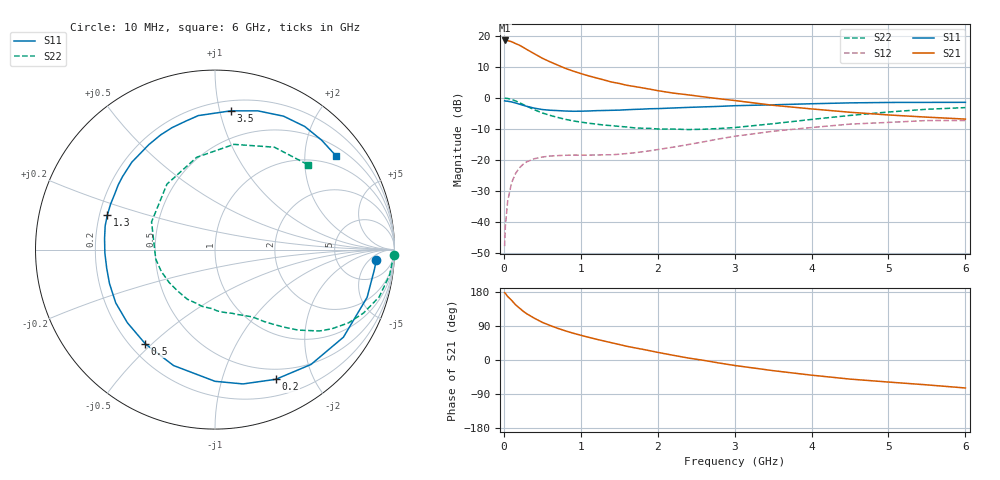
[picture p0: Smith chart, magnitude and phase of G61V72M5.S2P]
! SIEMENS Small Signal Semiconductors
! BFG193
! Si NPN RF Bipolar Junction Transistor in SOT223
! VCE = 1.75 V  IC = 2.5 mA
! Common Emitter S-Parameters:  August  1996
# GHz  S  MA  R  50
!  f  S11  S21  S12  S22
! GHz  MAG  ANG  MAG  ANG  MAG  ANG  MAG  ANG
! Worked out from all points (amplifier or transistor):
!   36 points, 10 MHz to 6 GHz, reference 50 ohm
!   highest |S21| = 18.6 dB at 10 MHz (marker M1)
!   |S21| within 3 dB of that: start of sweep to 305.1 MHz
!   unconditionally stable (mu >= 1): 1.312 GHz to 2.751 GHz
!   at 250 MHz: K = 0.21, MSG = 18.9 dB, |S12| = -21.4 dB
!   at 1.4 GHz: K = 1.07, MAG = 10.1 dB, |S12| = -18.3 dB
!   at 6 GHz: K = 0.97, MSG = 0.2 dB, |S12| = -7.2 dB
!   S11 on the Smith chart (normalised r, x): 10 MHz: 14, -8; 200 MHz: 0.38, -1.51; 500 MHz: 0.26, -0.48; 1.3 GHz: 0.23, +0.15; 3.5 GHz: 0.28, +1.08; 6 GHz: 0.72, +2.75
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0.01  0.9012 -3.6  8.472 177.5  0.0041 90.1  0.9951 -1.6
0.02  0.8948 -7.2  8.433 176.0  0.0086 87.0  0.9917 -3.3
0.05  0.8883 -17.4  8.411 167.6  0.0219 79.9  0.9832 -8.3
0.1  0.8661 -34.3  8.093 157.8  0.0428 72.1  0.9518 -16.1
0.15  0.8341 -50.1  7.578 146.1  0.0601 62.4  0.9 -23.1
0.2  0.798 -64.9  7.131 137.6  0.0744 56.0  0.8482 -28.8
0.25  0.7646 -78.2  6.582 128.9  0.0855 49.2  0.7867 -34.1
0.3  0.7338 -90.0  6.047 121.7  0.0941 44.6  0.7382 -37.9
0.4  0.686 -109.7  5.144 109.9  0.1055 36.5  0.6445 -44.1
0.5  0.6529 -126.5  4.382 99.4  0.112 30.3  0.5747 -48.6
0.6  0.6358 -140.2  3.838 91.1  0.1163 26.4  0.5257 -52.2
0.7  0.6277 -151.8  3.391 83.6  0.1181 23.7  0.4873 -55.5
0.9  0.6122 -170.3  2.722 70.8  0.1204 20.4  0.4283 -61.1
1.1  0.6183 174.3  2.28 60.0  0.1202 19.7  0.3934 -68.1
1.3  0.63 162.0  1.96 50.2  0.1218 20.2  0.3671 -75.0
1.6  0.6485 146.3  1.605 36.1  0.1276 22.8  0.3417 -88.0
2.2  0.6912 122.3  1.202 12.5  0.1617 26.4  0.3166 -119.2
2.8  0.7338 102.9  0.973 -8.0  0.2199 22.2  0.323 -157.8
3.5  0.7778 83.6  0.764 -28.1  0.2917 8.1  0.3858 156.4
4.5  0.8358 62.8  0.59 -50.4  0.3798 -14.1  0.5244 101.2
5.5  0.8512 45.8  0.492 -65.6  0.4339 -40.6  0.6596 59.9
6  0.8529 37.8  0.458 -73.9  0.435 -55.2  0.7012 42.4
